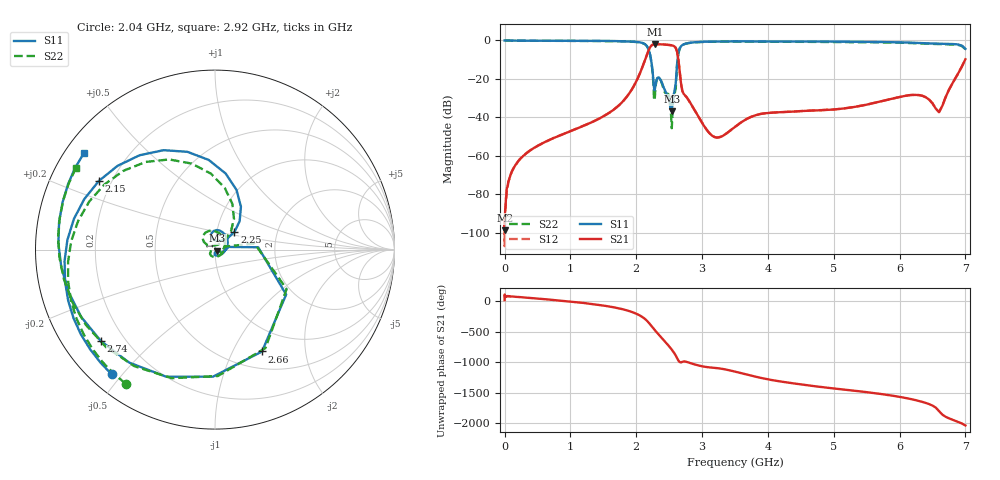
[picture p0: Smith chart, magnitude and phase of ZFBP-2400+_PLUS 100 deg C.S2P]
! Mini-Circuits
! S2P DATA File Format
! Type: BAND PASS FILTER
! Model: ZFBP-2400+
! All S Parameters are in dB deg format
! TEST CONDITIONS: INPUT POWER = 0 dBm @ Temperature = +100 deg C
! 401 Frequency points
# MHz S DB R 50
!FREQMAG(S11)PHS(S11)MAG(S21)PHS(S21)MAG(S12)PHS(S12)MAG(S22)PHS(S22)
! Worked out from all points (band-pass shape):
!   401 points, 500 kHz to 7 GHz, reference 50 ohm
!   highest |S21| = -1.92 dB at 2.29 GHz (marker M1); lowest = -98.8 dB at 2 MHz (marker M2)
!   |S21| within 3 dB of the highest: 2.19 GHz to 2.612 GHz (421.1 MHz wide, 17.5 % of centre)
!   lowest |S11| = -37.0 dB at 2.54 GHz (marker M3), VSWR 1.03, Z = 51.3 - j0.698 ohm
!   |S11| at or under -10 dB: 2.225 GHz to 2.628 GHz (403.5 MHz wide, 16.6 % of centre)
!   |S22| runs from -45.7 to 0.0 dB; largest |S21 - S12| = 0.0012
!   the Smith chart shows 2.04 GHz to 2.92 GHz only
!   S11 on the Smith chart (normalised r, x): 2.04 GHz: 0.06, -0.47; 2.15 GHz: 0.15, +0.27; 2.25 GHz: 1.22, +0.25; 2.66 GHz: 0.70, -1.31; 2.74 GHz: 0.11, -0.35; 2.92 GHz: 0.05, +0.33
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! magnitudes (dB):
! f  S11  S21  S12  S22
! 500 kHz  0.0  -97.4  -93.6  0.0
! 2 MHz  0.0  -98.8  -95.5  0.0
! 290 MHz  -0.1  -59.9  -59.8  -0.1
! 1.17 GHz  -0.2  -44.9  -44.9  -0.2
! 1.73 GHz  -0.3  -34.0  -34.0  -0.4
! 2.04 GHz  -0.9  -18.4  -18.4  -0.9
! 2.15 GHz  -2.5  -8.5  -8.5  -2.5
! 2.21 GHz  -7.4  -3.6  -3.6  -7.5
! 2.25 GHz  -16.7  -2.2  -2.2  -17.4
! 2.29 GHz  -23.9  -1.9  -1.9  -25.4
! 2.34 GHz  -19.2  -2.0  -2.0  -19.2
! 2.54 GHz  -37.0  -2.5  -2.5  -45.7
! 2.58 GHz  -26.6  -3.1  -3.1  -28.2
! 2.66 GHz  -4.1  -16.1  -16.1  -4.2
! 2.74 GHz  -1.8  -28.5  -28.5  -1.8
! 2.92 GHz  -0.9  -38.2  -38.3  -0.9
! 3.2 GHz  -0.5  -50.4  -50.4  -0.6
! 3.52 GHz  -0.4  -44.4  -44.4  -0.6
! 4.7 GHz  -0.6  -36.4  -36.5  -0.7
! 5.85 GHz  -0.8  -30.6  -30.6  -1.0
! 6.6 GHz  -1.7  -37.3  -37.3  -1.9
! 7 GHz  -4.3  -9.8  -9.8  -4.6
